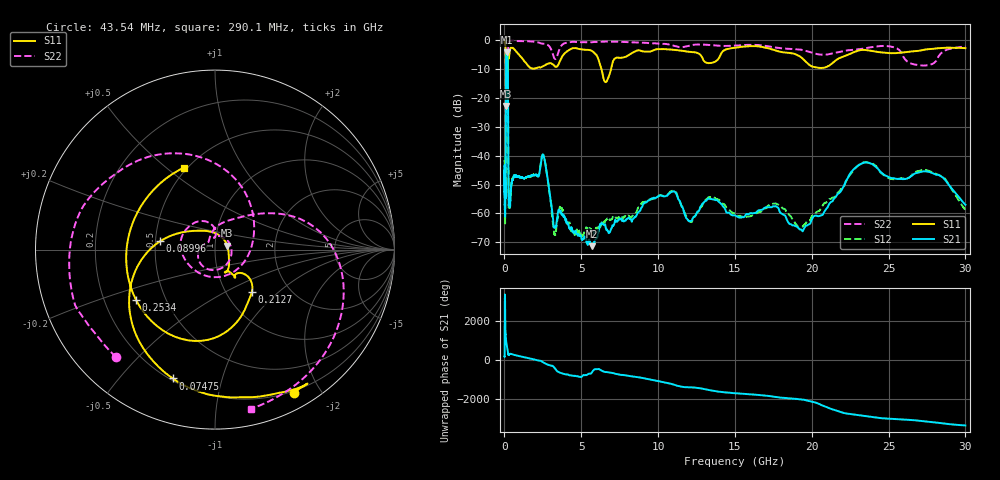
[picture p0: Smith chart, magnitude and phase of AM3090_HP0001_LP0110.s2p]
! Date/Time: Thu, Feb 28, 2019 1:54 PM
! Network Analyzer: Agilent Technologies E8364B Rev: A.07.50.67
! Sweep from 0.010 to 30.000 GHz, 1601 Points, Sweep Type: LOG
! Power Supply: 5.022 V, 0.002 A
# Hz S DB R 50
!freq MagS11 AngS11 MagS21 AngS21 MagS12 AngS12 MagS22 AngS22
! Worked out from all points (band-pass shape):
!   1601 points, 10 MHz to 30 GHz, reference 50 ohm
!   highest |S21| = -4.25 dB at 146.9 MHz (marker M1); lowest = -71.3 dB at 5.697 GHz (marker M2)
!   |S21| within 3 dB of the highest: 100 MHz to 210.3 MHz (110.3 MHz wide, 71.1 % of centre)
!   lowest |S11| = -22.9 dB at 98.44 MHz (marker M3), VSWR 1.16, Z = 57.3 + j2.47 ohm
!   |S11| at or under -10 dB: 89.85 MHz to 213.3 MHz (123.4 MHz wide, 81.4 % of centre); 6.308 GHz to 6.937 GHz (629.2 MHz wide, 9.5 % of centre)
!   |S22| runs from -25.1 to -0.2 dB; largest |S21 - S12| = 0.013
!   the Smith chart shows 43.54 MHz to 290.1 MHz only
!   S11 on the Smith chart (normalised r, x): 43.54 MHz: 0.18, -1.68; 74.75 MHz: 0.21, -0.70; 89.96 MHz: 0.53, +0.05; 212.7 MHz: 1.31, -0.69; 253.4 MHz: 0.34, -0.26; 290.1 MHz: 0.48, +0.57
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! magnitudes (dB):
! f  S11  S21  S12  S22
! 10 MHz  -0.3  -45.1  -42.0  -0.6
! 38.04 MHz  -0.5  -57.8  -61.2  -1.4
! 43.54 MHz  -0.8  -60.2  -60.5  -1.8
! 74.75 MHz  -2.4  -46.2  -45.6  -4.4
! 89.96 MHz  -10.2  -15.3  -15.3  -16.1
! 98.44 MHz  -22.9  -7.8  -7.8  -14.1
! 144.7 MHz  -15.3  -4.3  -4.2  -21.1
! 146.9 MHz  -15.2  -4.2  -4.2  -20.9
! 212.7 MHz  -10.1  -7.7  -7.7  -16.4
! 253.4 MHz  -5.7  -47.6  -46.7  -1.9
! 290.1 MHz  -6.2  -55.5  -57.9  -0.8
! 550.5 MHz  -2.8  -48.2  -47.7  -0.3
! 2.084 GHz  -9.8  -46.6  -46.9  -0.7
! 2.533 GHz  -9.0  -39.8  -39.7  -1.3
! 3.253 GHz  -9.0  -65.0  -67.4  -6.4
! 5.697 GHz  -3.8  -71.3  -66.1  -0.8
! 6.619 GHz  -14.5  -65.6  -62.2  -0.6
! 7.926 GHz  -5.7  -62.1  -61.1  -0.7
! 10.81 GHz  -3.3  -52.7  -52.4  -1.7
! 19.22 GHz  -5.7  -65.5  -64.5  -3.3
! 23.48 GHz  -3.5  -42.4  -42.3  -2.9
! 30 GHz  -2.8  -57.0  -58.8  -2.3
